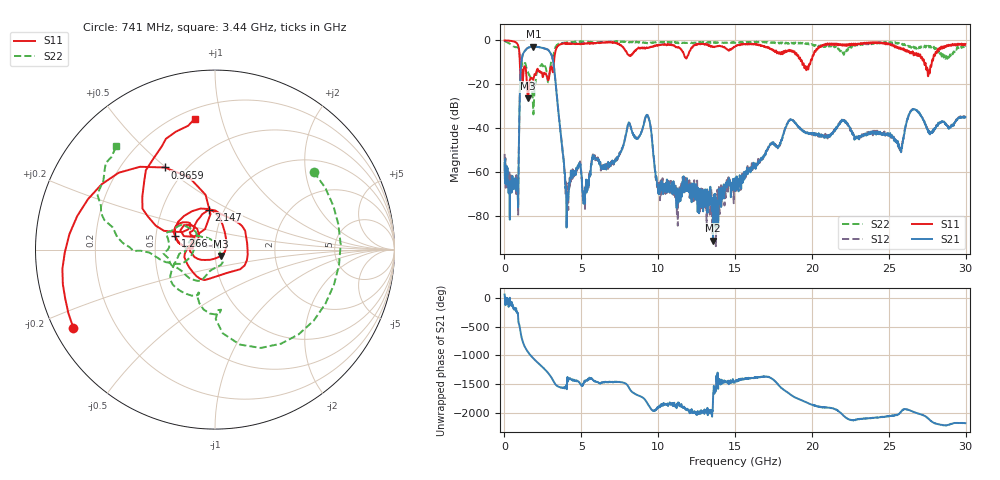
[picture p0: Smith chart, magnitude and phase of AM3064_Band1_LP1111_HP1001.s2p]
# Hz S DB R 50.0
!freq dBS11 angS11 dBS21 angS21 dBS12 angS12 dBS22 angS22
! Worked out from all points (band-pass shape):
!   1600 points, 10 MHz to 29.98 GHz, reference 50 ohm
!   highest |S21| = -2.82 dB at 1.884 GHz (marker M1); lowest = -91.2 dB at 13.56 GHz (marker M2)
!   |S21| within 3 dB of the highest: 1.233 GHz to 2.999 GHz (1.767 GHz wide, 83.5 % of centre)
!   lowest |S11| = -26.3 dB at 1.528 GHz (marker M3), VSWR 1.10, Z = 53.2 - j3.82 ohm
!   |S11| at or under -10 dB: 1.002 GHz to 3.22 GHz (2.218 GHz wide, 105 % of centre); 19.36 GHz to 19.91 GHz (545.3 MHz wide, 2.78 % of centre); 27.3 GHz to 27.8 GHz (496.5 MHz wide, 1.8 % of centre)
!   |S22| runs from -33.7 to -0.2 dB; largest |S21 - S12| = 0.013
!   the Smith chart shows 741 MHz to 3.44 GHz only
!   S11 on the Smith chart (normalised r, x): 741 MHz: 0.06, -0.26; 965.9 MHz: 0.39, +0.50; 1.266 GHz: 0.63, +0.10; 2.147 GHz: 0.85, +0.40; 3.44 GHz: 0.26, +0.82
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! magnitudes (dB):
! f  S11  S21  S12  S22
! 10 MHz  0.0  -55.7  -51.7  -0.2
! 741 MHz  -0.9  -63.9  -68.0  -3.1
! 965.9 MHz  -5.4  -36.2  -36.2  -5.2
! 1.266 GHz  -12.6  -5.4  -5.4  -10.8
! 1.528 GHz  -26.3  -3.4  -3.4  -14.5
! 1.884 GHz  -17.7  -2.8  -2.8  -33.7
! 2.147 GHz  -12.9  -3.1  -3.0  -13.7
! 3.046 GHz  -11.9  -6.4  -6.4  -9.7
! 3.44 GHz  -2.7  -27.7  -27.4  -2.0
! 4.059 GHz  -1.2  -79.5  -74.4  -0.9
! 5.015 GHz  -1.5  -61.4  -62.9  -0.5
! 9.288 GHz  -3.5  -33.9  -34.0  -1.4
! 10 GHz  -2.2  -67.2  -65.3  -0.9
! 13.56 GHz  -2.9  -91.2  -72.8  -1.1
! 15 GHz  -2.8  -68.6  -65.9  -1.2
! 18.57 GHz  -5.0  -36.5  -36.2  -1.2
! 19.99 GHz  -8.9  -42.6  -42.5  -1.7
! 25 GHz  -1.4  -42.6  -42.5  -1.1
! 25.76 GHz  -3.9  -50.3  -50.2  -1.3
! 26.61 GHz  -6.7  -31.4  -31.4  -2.9
! 27.56 GHz  -16.4  -41.9  -41.4  -2.6
! 29.98 GHz  -1.7  -34.9  -34.8  -2.9
